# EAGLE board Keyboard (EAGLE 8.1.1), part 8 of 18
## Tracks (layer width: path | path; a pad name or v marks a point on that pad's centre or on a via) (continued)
S$7677 (continued)
  Bottom 0: 271.1,39.77 271.09,39.71
S$7678
  Bottom 0: 271.09,39.71 271.09,39.64
S$7679
  Bottom 0: 271.09,39.64 271.09,38.2
S$7680
  Bottom 0: 271.09,38.2 268.72,38.2
S$7681
  Bottom 0: 268.72,38.2 268.71,38.22
S$7682
  Bottom 0: 268.71,38.22 268.5,38.38
S$7683
  Bottom 0: 268.5,38.38 268.26,38.44
S$7684
  Bottom 0: 268.26,38.44 268.01,38.42
S$7685
  Bottom 0: 268.01,38.42 267.79,38.31
S$7686
  Bottom 0: 267.79,38.31 267.61,38.12
S$7687
  Bottom 0: 267.61,38.12 267.53,37.89
S$7688
  Bottom 0: 267.53,37.89 267.53,37.63
S$7689
  Bottom 0: 267.53,37.63 267.61,37.4
S$7690
  Bottom 0: 267.61,37.4 267.79,37.21
S$7691
  Bottom 0: 267.79,37.21 268.01,37.1
S$7692
  Bottom 0: 268.01,37.1 268.26,37.08
S$7693
  Bottom 0: 268.26,37.08 268.5,37.15
S$7694
  Bottom 0: 268.5,37.15 268.71,37.3
S$7695
  Bottom 0: 268.71,37.3 268.72,37.32
S$7696
  Bottom 0: 268.72,37.32 271.09,37.32
S$7697
  Bottom 0: 271.09,37.32 271.09,15.75
S$7698
  Bottom 0: 271.09,15.75 271.09,15.68
S$7699
  Bottom 0: 271.09,15.68 271.1,15.61
S$7700
  Bottom 0: 271.1,15.61 271.13,15.55
S$7701
  Bottom 0: 271.13,15.55 271.17,15.49
S$7702
  Bottom 0: 271.17,15.49 271.21,15.44
S$7703
  Bottom 0: 271.21,15.44 276.79,9.86
S$7704
  Bottom 0: 276.79,9.86 276.84,9.82
S$7705
  Bottom 0: 276.84,9.82 276.9,9.78
S$7706
  Bottom 0: 276.9,9.78 276.96,9.76
S$7707
  Bottom 0: 276.96,9.76 277.03,9.74
S$7708
  Bottom 0: 277.03,9.74 277.1,9.74
S$7709
  Bottom 0: 277.1,9.74 277.62,9.74
S$7710
  Bottom 0: 277.62,9.74 277.37,9.66
S$7711
  Bottom 0: 277.37,9.66 276.97,9.45
S$7712
  Bottom 0: 276.97,9.45 276.62,9.16
S$7713
  Bottom 0: 276.62,9.16 276.34,8.82
S$7714
  Bottom 0: 276.34,8.82 276.12,8.42
S$7715
  Bottom 0: 276.12,8.42 276,7.99
S$7716
  Bottom 0: 276,7.99 275.95,7.55
S$7717
  Bottom 0: 275.95,7.55 276,7.1
S$7718
  Bottom 0: 276,7.1 276.11,6.75
S$7719
  Bottom 0: 107.77,7.27 107.8,7.43
S$7720
  Bottom 0: 107.8,7.43 107.75,7.75
S$7721
  Bottom 0: 107.75,7.75 107.75,7.78
S$7722
  Bottom 0: 107.75,7.78 107.88,7.9
S$7723
  Bottom 0: 107.88,7.9 107.94,7.97
S$7724
  Bottom 0: 107.94,7.97 107.98,8.04
S$7725
  Bottom 0: 107.98,8.04 108.02,8.12
S$7726
  Bottom 0: 108.02,8.12 108.04,8.21
S$7727
  Bottom 0: 108.04,8.21 108.04,8.3
S$7728
  Bottom 0: 108.04,8.3 108.04,22.57
S$7729
  Bottom 0: 108.04,22.57 108.08,22.6
S$7730
  Bottom 0: 108.08,22.6 110.11,24.64
S$7731
  Bottom 0: 110.11,24.64 110.08,24.58
S$7732
  Bottom 0: 110.08,24.58 109.99,24.24
S$7733
  Bottom 0: 109.99,24.24 109.99,23.89
S$7734
  Bottom 0: 109.99,23.89 110.08,23.55
S$7735
  Bottom 0: 110.08,23.55 110.25,23.24
S$7736
  Bottom 0: 110.25,23.24 110.49,22.99
S$7737
  Bottom 0: 110.49,22.99 110.78,22.8
S$7738
  Bottom 0: 110.78,22.8 110.94,22.75
S$7739
  Bottom 0: 110.94,22.75 110.94,10.43
S$7740
  Bottom 0: 110.94,10.43 107.77,7.27
S$7741
  Bottom 0: 45.16,10.87 45.31,11.02
S$7742
  Bottom 0: 45.31,11.02 45.44,11.29
S$7743
  Bottom 0: 45.44,11.29 45.48,11.6
S$7744
  Bottom 0: 45.48,11.6 45.44,11.89
S$7745
  Bottom 0: 45.44,11.89 45.31,12.17
S$7746
  Bottom 0: 45.31,12.17 45.1,12.39
S$7747
  Bottom 0: 45.1,12.39 44.84,12.54
S$7748
  Bottom 0: 44.84,12.54 44.54,12.61
S$7749
  Bottom 0: 44.54,12.61 44.24,12.59
S$7750
  Bottom 0: 44.24,12.59 44.14,12.55
S$7751
  Bottom 0: 44.14,12.55 43.71,12.99
S$7752
  Bottom 0: 43.71,12.99 43.65,13.03
S$7753
  Bottom 0: 43.65,13.03 43.59,13.07
S$7754
  Bottom 0: 43.59,13.07 43.53,13.09
S$7755
  Bottom 0: 43.53,13.09 43.46,13.11
S$7756
  Bottom 0: 43.46,13.11 43.39,13.11
S$7757
  Bottom 0: 43.39,13.11 37.02,13.11
S$7758
  Bottom 0: 37.02,13.11 36.94,13.11
S$7759
  Bottom 0: 36.94,13.11 36.88,13.09
S$7760
  Bottom 0: 36.88,13.09 36.82,13.07
S$7761
  Bottom 0: 36.82,13.07 36.76,13.03
S$7762
  Bottom 0: 36.76,13.03 36.7,12.99
S$7763
  Bottom 0: 36.7,12.99 36.13,12.42
S$7764
  Bottom 0: 36.13,12.42 36.16,12.64
S$7765
  Bottom 0: 36.16,12.64 36.12,12.96
S$7766
  Bottom 0: 36.12,12.96 35.98,13.26
S$7767
  Bottom 0: 35.98,13.26 35.77,13.5
S$7768
  Bottom 0: 35.77,13.5 35.59,13.62
S$7769
  Bottom 0: 35.59,13.62 35.59,16.83
S$7770
  Bottom 0: 35.59,16.83 53.03,16.83
S$7771
  Bottom 0: 53.03,16.83 52.84,16.64
S$7772
  Bottom 0: 52.84,16.64 52.66,16.36
S$7773
  Bottom 0: 52.66,16.36 52.58,16.05
S$7774
  Bottom 0: 52.58,16.05 52.58,15.72
S$7775
  Bottom 0: 52.58,15.72 52.66,15.41
S$7776
  Bottom 0: 52.66,15.41 52.84,15.14
S$7777
  Bottom 0: 52.84,15.14 53.07,14.91
S$7778
  Bottom 0: 53.07,14.91 53.36,14.77
S$7779
  Bottom 0: 53.36,14.77 53.68,14.7
S$7780
  Bottom 0: 53.68,14.7 54,14.72
S$7781
  Bottom 0: 54,14.72 54.22,14.8
S$7782
  Bottom 0: 54.22,14.8 55.28,13.74
S$7783
  Bottom 0: 55.28,13.74 55.26,13.73
S$7784
  Bottom 0: 55.26,13.73 55.2,13.67
S$7785
  Bottom 0: 55.2,13.67 55.16,13.6
S$7786
  Bottom 0: 55.16,13.6 55.15,13.53
S$7787
  Bottom 0: 55.15,13.53 55.15,11.75
S$7788
  Bottom 0: 55.15,11.75 55.16,11.67
S$7789
  Bottom 0: 55.16,11.67 55.2,11.6
S$7790
  Bottom 0: 55.2,11.6 55.26,11.54
S$7791
  Bottom 0: 55.26,11.54 55.33,11.5
S$7792
  Bottom 0: 55.33,11.5 55.41,11.49
S$7793
  Bottom 0: 55.41,11.49 57.18,11.49
S$7794
  Bottom 0: 57.18,11.49 57.26,11.5
S$7795
  Bottom 0: 57.26,11.5 57.33,11.54
S$7796
  Bottom 0: 57.33,11.54 57.38,11.6
S$7797
  Bottom 0: 57.38,11.6 57.43,11.67
S$7798
  Bottom 0: 57.43,11.67 57.44,11.75
S$7799
  Bottom 0: 57.44,11.75 57.44,13.23
S$7800
  Bottom 0: 57.44,13.23 57.73,12.94
S$7801
  Bottom 0: 57.73,12.94 57.69,12.64
S$7802
  Bottom 0: 57.69,12.64 57.73,12.32
S$7803
  Bottom 0: 57.73,12.32 57.87,12.02
S$7804
  Bottom 0: 57.87,12.02 58.09,11.77
S$7805
  Bottom 0: 58.09,11.77 58.36,11.6
S$7806
  Bottom 0: 58.36,11.6 58.67,11.5
S$7807
  Bottom 0: 58.67,11.5 58.96,11.5
S$7808
  Bottom 0: 58.96,11.5 58.32,10.87
S$7809
  Bottom 0: 58.32,10.87 49.93,10.87
S$7810
  Bottom 0: 49.93,10.87 50.07,11.02
S$7811
  Bottom 0: 50.07,11.02 50.2,11.29
S$7812
  Bottom 0: 50.2,11.29 50.25,11.6
S$7813
  Bottom 0: 50.25,11.6 50.2,11.89
S$7814
  Bottom 0: 50.2,11.89 50.07,12.17
S$7815
  Bottom 0: 50.07,12.17 49.87,12.39
S$7816
  Bottom 0: 49.87,12.39 49.6,12.54
S$7817
  Bottom 0: 49.6,12.54 49.31,12.61
S$7818
  Bottom 0: 49.31,12.61 49,12.59
S$7819
  Bottom 0: 49,12.59 48.73,12.47
S$7820
  Bottom 0: 48.73,12.47 48.49,12.29
S$7821
  Bottom 0: 48.49,12.29 48.32,12.04
S$7822
  Bottom 0: 48.32,12.04 48.23,11.75
S$7823
  Bottom 0: 48.23,11.75 48.23,11.44
S$7824
  Bottom 0: 48.23,11.44 48.32,11.15
S$7825
  Bottom 0: 48.32,11.15 48.49,10.9
S$7826
  Bottom 0: 48.49,10.9 48.53,10.87
S$7827
  Bottom 0: 48.53,10.87 45.16,10.87
S$7828
  Bottom 0: 288.12,10.9 288.22,11.02
S$7829
  Bottom 0: 288.22,11.02 288.35,11.29
S$7830
  Bottom 0: 288.35,11.29 288.4,11.6
S$7831
  Bottom 0: 288.4,11.6 288.35,11.89
S$7832
  Bottom 0: 288.35,11.89 288.22,12.17
S$7833
  Bottom 0: 288.22,12.17 288.02,12.39
S$7834
  Bottom 0: 288.02,12.39 287.75,12.54
S$7835
  Bottom 0: 287.75,12.54 287.46,12.61
S$7836
  Bottom 0: 287.46,12.61 287.15,12.59
S$7837
  Bottom 0: 287.15,12.59 286.98,12.52
S$7838
  Bottom 0: 286.98,12.52 287.69,13.23
S$7839
  Bottom 0: 287.69,13.23 287.75,13.29
S$7840
  Bottom 0: 287.75,13.29 287.8,13.37
S$7841
  Bottom 0: 287.8,13.37 287.83,13.45
S$7842
  Bottom 0: 287.83,13.45 287.85,13.54
S$7843
  Bottom 0: 287.85,13.54 287.86,13.63
S$7844
  Bottom 0: 287.86,13.63 287.86,22.31
S$7845
  Bottom 0: 287.86,22.31 288.06,22.15
S$7846
  Bottom 0: 288.06,22.15 288.34,22.04
S$7847
  Bottom 0: 288.34,22.04 288.64,22.02
S$7848
  Bottom 0: 288.64,22.02 288.89,22.07
S$7849
  Bottom 0: 288.89,22.07 289.77,21.2
S$7850
  Bottom 0: 289.77,21.2 289.83,21.15
S$7851
  Bottom 0: 289.83,21.15 289.88,21.11
S$7852
  Bottom 0: 289.88,21.11 289.95,21.09
S$7853
  Bottom 0: 289.95,21.09 290.01,21.07
S$7854
  Bottom 0: 290.01,21.07 290.09,21.06
S$7855
  Bottom 0: 290.09,21.06 293.43,21.06
S$7856
  Bottom 0: 293.43,21.06 293.45,20.99
S$7857
  Bottom 0: 293.45,20.99 293.63,20.68
S$7858
  Bottom 0: 293.63,20.68 293.87,20.43
S$7859
  Bottom 0: 293.87,20.43 294.16,20.24
S$7860
  Bottom 0: 294.16,20.24 294.49,20.14
S$7861
  Bottom 0: 294.49,20.14 294.84,20.11
S$7862
  Bottom 0: 294.84,20.11 295.14,20.17
S$7863
  Bottom 0: 295.14,20.17 295.25,20.14
S$7864
  Bottom 0: 295.25,20.14 295.6,20.11
S$7865
  Bottom 0: 295.6,20.11 295.71,20.14
S$7866
  Bottom 0: 295.71,20.14 289.45,13.87
S$7867
  Bottom 0: 289.45,13.87 289.4,13.81
S$7868
  Bottom 0: 289.4,13.81 289.36,13.75
S$7869
  Bottom 0: 289.36,13.75 289.34,13.69
S$7870
  Bottom 0: 289.34,13.69 289.32,13.63
S$7871
  Bottom 0: 289.32,13.63 289.32,13.56
S$7872
  Bottom 0: 289.32,13.56 289.32,12.5
S$7873
  Bottom 0: 289.32,12.5 289.25,12.47
S$7874
  Bottom 0: 289.25,12.47 289.01,12.29
S$7875
  Bottom 0: 289.01,12.29 288.85,12.04
S$7876
  Bottom 0: 288.85,12.04 288.75,11.75
S$7877
  Bottom 0: 288.75,11.75 288.75,11.44
S$7878
  Bottom 0: 288.75,11.44 288.85,11.15
S$7879
  Bottom 0: 288.85,11.15 289.01,10.9
S$7880
  Bottom 0: 289.01,10.9 288.12,10.9
S$7881
  Bottom 0: 290.49,10.9 290.6,11.02
S$7882
  Bottom 0: 290.6,11.02 290.73,11.29
S$7883
  Bottom 0: 290.73,11.29 290.78,11.6
S$7884
  Bottom 0: 290.78,11.6 290.73,11.89
S$7885
  Bottom 0: 290.73,11.89 290.6,12.17
S$7886
  Bottom 0: 290.6,12.17 290.4,12.39
S$7887
  Bottom 0: 290.4,12.39 290.2,12.5
S$7888
  Bottom 0: 290.2,12.5 290.2,13.37
S$7889
  Bottom 0: 290.2,13.37 293.19,16.36
S$7890
  Bottom 0: 293.19,16.36 293.11,16.05
S$7891
  Bottom 0: 293.11,16.05 293.11,15.72
S$7892
  Bottom 0: 293.11,15.72 293.19,15.41
S$7893
  Bottom 0: 293.19,15.41 293.37,15.14
S$7894
  Bottom 0: 293.37,15.14 293.6,14.91
S$7895
  Bottom 0: 293.6,14.91 293.89,14.77
S$7896
  Bottom 0: 293.89,14.77 294.21,14.7
S$7897
  Bottom 0: 294.21,14.7 294.53,14.72
S$7898
  Bottom 0: 294.53,14.72 294.57,14.73
S$7899
  Bottom 0: 294.57,14.73 295.52,13.77
S$7900
  Bottom 0: 295.52,13.77 295.13,13.77
S$7901
  Bottom 0: 295.13,13.77 295.06,13.76
S$7902
  Bottom 0: 295.06,13.76 294.99,13.72
S$7903
  Bottom 0: 294.99,13.72 294.93,13.66
S$7904
  Bottom 0: 294.93,13.66 294.89,13.59
S$7905
  Bottom 0: 294.89,13.59 294.88,13.52
S$7906
  Bottom 0: 294.88,13.52 294.88,11.74
S$7907
  Bottom 0: 294.88,11.74 294.89,11.66
S$7908
  Bottom 0: 294.89,11.66 294.93,11.59
S$7909
  Bottom 0: 294.93,11.59 294.99,11.53
S$7910
  Bottom 0: 294.99,11.53 295.06,11.49
S$7911
  Bottom 0: 295.06,11.49 295.13,11.48
S$7912
  Bottom 0: 295.13,11.48 297.19,11.48
S$7913
  Bottom 0: 297.19,11.48 296.61,10.9
S$7914
  Bottom 0: 296.61,10.9 290.49,10.9
S$7915
  Bottom 0: 219.65,11.68 207.87,23.45
S$7916
  Bottom 0: 207.87,23.45 207.98,23.72
S$7917
  Bottom 0: 207.98,23.72 208.02,24.07
S$7918
  Bottom 0: 208.02,24.07 207.98,24.41
S$7919
  Bottom 0: 207.98,24.41 207.87,24.69
S$7920
  Bottom 0: 207.87,24.69 208.32,25.14
S$7921
  Bottom 0: 208.32,25.14 208.36,25.19
S$7922
  Bottom 0: 208.36,25.19 208.4,25.25
S$7923
  Bottom 0: 208.4,25.25 208.43,25.32
S$7924
  Bottom 0: 208.43,25.32 208.44,25.38
S$7925
  Bottom 0: 208.44,25.38 208.45,25.45
S$7926
  Bottom 0: 208.45,25.45 208.45,40.27
S$7927
  Bottom 0: 208.45,40.27 208.5,40.06
S$7928
  Bottom 0: 208.5,40.06 208.67,39.75
S$7929
  Bottom 0: 208.67,39.75 208.91,39.5
S$7930
  Bottom 0: 208.91,39.5 209.21,39.31
S$7931
  Bottom 0: 209.21,39.31 209.54,39.2
S$7932
  Bottom 0: 209.54,39.2 209.89,39.19
S$7933
  Bottom 0: 209.89,39.19 210.23,39.25
S$7934
  Bottom 0: 210.23,39.25 210.55,39.4
S$7935
  Bottom 0: 210.55,39.4 210.82,39.62
S$7936
  Bottom 0: 210.82,39.62 211.03,39.91
S$7937
  Bottom 0: 211.03,39.91 211.15,40.23
S$7938
  Bottom 0: 211.15,40.23 211.2,40.58
S$7939
  Bottom 0: 211.2,40.58 211.15,40.92
S$7940
  Bottom 0: 211.15,40.92 211.03,41.25
S$7941
  Bottom 0: 211.03,41.25 210.82,41.53
S$7942
  Bottom 0: 210.82,41.53 210.55,41.76
S$7943
  Bottom 0: 210.55,41.76 210.23,41.91
S$7944
  Bottom 0: 210.23,41.91 209.89,41.97
S$7945
  Bottom 0: 209.89,41.97 209.54,41.95
S$7946
  Bottom 0: 209.54,41.95 209.21,41.84
S$7947
  Bottom 0: 209.21,41.84 208.91,41.65
S$7948
  Bottom 0: 208.91,41.65 208.67,41.4
S$7949
  Bottom 0: 208.67,41.4 208.5,41.09
S$7950
  Bottom 0: 208.5,41.09 208.45,40.89
S$7951
  Bottom 0: 208.45,40.89 208.45,41.26
S$7952
  Bottom 0: 208.45,41.26 208.44,41.33
S$7953
  Bottom 0: 208.44,41.33 208.43,41.39
S$7954
  Bottom 0: 208.43,41.39 208.4,41.45
S$7955
  Bottom 0: 208.4,41.45 208.36,41.52
S$7956
  Bottom 0: 208.36,41.52 208.32,41.57
S$7957
  Bottom 0: 208.32,41.57 201.82,48.08
S$7958
  Bottom 0: 201.82,48.08 201.83,48.12
S$7959
  Bottom 0: 201.83,48.12 201.78,48.37
S$7960
  Bottom 0: 201.78,48.37 201.65,48.59
S$7961
  Bottom 0: 201.65,48.59 201.45,48.74
S$7962
  Bottom 0: 201.45,48.74 201.21,48.81
S$7963
  Bottom 0: 201.21,48.81 200.96,48.78
S$7964
  Bottom 0: 200.96,48.78 200.73,48.67
S$7965
  Bottom 0: 200.73,48.67 200.56,48.49
S$7966
  Bottom 0: 200.56,48.49 200.47,48.25
S$7967
  Bottom 0: 200.47,48.25 200.47,48.18
S$7968
  Bottom 0: 200.47,48.18 196.29,52.36
S$7969
  Bottom 0: 196.29,52.36 196.79,52.85
S$7970
  Bottom 0: 196.79,52.85 197.04,52.8
S$7971
  Bottom 0: 197.04,52.8 197.37,52.82
S$7972
  Bottom 0: 197.37,52.82 197.67,52.93
S$7973
  Bottom 0: 197.67,52.93 197.94,53.11
S$7974
  Bottom 0: 197.94,53.11 198.14,53.37
S$7975
  Bottom 0: 198.14,53.37 198.27,53.67
S$7976
  Bottom 0: 198.27,53.67 198.32,53.98
S$7977
  Bottom 0: 198.32,53.98 198.27,54.3
S$7978
  Bottom 0: 198.27,54.3 198.14,54.61
S$7979
  Bottom 0: 198.14,54.61 197.94,54.86
S$7980
  Bottom 0: 197.94,54.86 197.67,55.05
S$7981
  Bottom 0: 197.67,55.05 197.37,55.16
S$7982
  Bottom 0: 197.37,55.16 197.04,55.18
S$7983
  Bottom 0: 197.04,55.18 196.72,55.11
S$7984
  Bottom 0: 196.72,55.11 196.43,54.96
S$7985
  Bottom 0: 196.43,54.96 196.2,54.74
S$7986
  Bottom 0: 196.2,54.74 196.02,54.47
S$7987
  Bottom 0: 196.02,54.47 195.94,54.15
S$7988
  Bottom 0: 195.94,54.15 195.94,53.83
S$7989
  Bottom 0: 195.94,53.83 195.98,53.66
S$7990
  Bottom 0: 195.98,53.66 195.25,52.93
S$7991
  Bottom 0: 195.25,52.93 190.05,52.93
S$7992
  Bottom 0: 190.05,52.93 190.31,53.11
S$7993
  Bottom 0: 190.31,53.11 190.52,53.37
S$7994
  Bottom 0: 190.52,53.37 190.65,53.67
S$7995
  Bottom 0: 190.65,53.67 190.7,53.98
S$7996
  Bottom 0: 190.7,53.98 190.65,54.3
S$7997
  Bottom 0: 190.65,54.3 190.52,54.61
S$7998
  Bottom 0: 190.52,54.61 190.31,54.86
S$7999
  Bottom 0: 190.31,54.86 190.05,55.05
S$8000
  Bottom 0: 190.05,55.05 189.75,55.16
S$8001
  Bottom 0: 189.75,55.16 189.42,55.18
S$8002
  Bottom 0: 189.42,55.18 189.1,55.11
S$8003
  Bottom 0: 189.1,55.11 188.81,54.96
S$8004
  Bottom 0: 188.81,54.96 188.58,54.74
S$8005
  Bottom 0: 188.58,54.74 188.41,54.47
S$8006
  Bottom 0: 188.41,54.47 188.32,54.15
S$8007
  Bottom 0: 188.32,54.15 188.32,53.83
S$8008
  Bottom 0: 188.32,53.83 188.41,53.51
S$8009
  Bottom 0: 188.41,53.51 188.58,53.23
S$8010
  Bottom 0: 188.58,53.23 188.81,53.01
S$8011
  Bottom 0: 188.81,53.01 188.98,52.93
S$8012
  Bottom 0: 188.98,52.93 179.94,52.93
S$8013
  Bottom 0: 179.94,52.93 179.22,53.65
S$8014
  Bottom 0: 179.22,53.65 179.22,53.67
S$8015
  Bottom 0: 179.22,53.67 179.27,53.98
S$8016
  Bottom 0: 179.27,53.98 179.22,54.3
S$8017
  Bottom 0: 179.22,54.3 179.09,54.61
S$8018
  Bottom 0: 179.09,54.61 178.88,54.86
S$8019
  Bottom 0: 178.88,54.86 178.62,55.05
S$8020
  Bottom 0: 178.62,55.05 178.32,55.16
S$8021
  Bottom 0: 178.32,55.16 177.99,55.18
S$8022
  Bottom 0: 177.99,55.18 177.67,55.11
S$8023
  Bottom 0: 177.67,55.11 177.38,54.96
S$8024
  Bottom 0: 177.38,54.96 177.15,54.74
S$8025
  Bottom 0: 177.15,54.74 176.97,54.47
S$8026
  Bottom 0: 176.97,54.47 176.89,54.15
S$8027
  Bottom 0: 176.89,54.15 176.89,53.83
S$8028
  Bottom 0: 176.89,53.83 176.97,53.51
S$8029
  Bottom 0: 176.97,53.51 177.15,53.23
S$8030
  Bottom 0: 177.15,53.23 177.38,53.01
S$8031
  Bottom 0: 177.38,53.01 177.67,52.87
S$8032
  Bottom 0: 177.67,52.87 177.99,52.8
S$8033
  Bottom 0: 177.99,52.8 178.32,52.82
S$8034
  Bottom 0: 178.32,52.82 178.41,52.85
S$8035
  Bottom 0: 178.41,52.85 179.14,52.12
S$8036
  Bottom 0: 179.14,52.12 179.14,43.98
S$8037
  Bottom 0: 179.14,43.98 179.07,44.07
S$8038
  Bottom 0: 179.07,44.07 178.8,44.3
S$8039
  Bottom 0: 178.8,44.3 178.49,44.44
S$8040
  Bottom 0: 178.49,44.44 178.49,50.68
S$8041
  Bottom 0: 178.49,50.68 178.49,50.75
S$8042
  Bottom 0: 178.49,50.75 178.47,50.81
S$8043
  Bottom 0: 178.47,50.81 178.45,50.87
S$8044
  Bottom 0: 178.45,50.87 178.41,50.94
S$8045
  Bottom 0: 178.41,50.94 178.37,50.99
S$8046
  Bottom 0: 178.37,50.99 173.39,55.96
S$8047
  Bottom 0: 173.39,55.96 173.4,56.01
S$8048
  Bottom 0: 173.4,56.01 173.36,56.26
S$8049
  Bottom 0: 173.36,56.26 173.22,56.47
S$8050
  Bottom 0: 173.22,56.47 173.02,56.62
S$8051
  Bottom 0: 173.02,56.62 172.78,56.69
S$8052
  Bottom 0: 172.78,56.69 172.53,56.67
S$8053
  Bottom 0: 172.53,56.67 172.3,56.56
S$8054
  Bottom 0: 172.3,56.56 172.13,56.37
S$8055
  Bottom 0: 172.13,56.37 172.04,56.14
S$8056
  Bottom 0: 172.04,56.14 172.04,55.88
S$8057
  Bottom 0: 172.04,55.88 172.13,55.65
S$8058
  Bottom 0: 172.13,55.65 172.3,55.46
S$8059
  Bottom 0: 172.3,55.46 172.53,55.35
S$8060
  Bottom 0: 172.53,55.35 172.77,55.33
S$8061
  Bottom 0: 172.77,55.33 177.61,50.49
S$8062
  Bottom 0: 177.61,50.49 177.61,44.43
S$8063
  Bottom 0: 177.61,44.43 177.46,44.38
S$8064
  Bottom 0: 177.46,44.38 177.16,44.19
S$8065
  Bottom 0: 177.16,44.19 176.92,43.94
S$8066
  Bottom 0: 176.92,43.94 176.75,43.63
S$8067
  Bottom 0: 176.75,43.63 176.66,43.29
S$8068
  Bottom 0: 176.66,43.29 176.66,42.94
S$8069
  Bottom 0: 176.66,42.94 176.75,42.6
S$8070
  Bottom 0: 176.75,42.6 176.92,42.29
S$8071
  Bottom 0: 176.92,42.29 177.16,42.04
S$8072
  Bottom 0: 177.16,42.04 177.46,41.85
S$8073
  Bottom 0: 177.46,41.85 177.79,41.74
S$8074
  Bottom 0: 177.79,41.74 178.14,41.73
S$8075
  Bottom 0: 178.14,41.73 178.48,41.79
S$8076
  Bottom 0: 178.48,41.79 178.8,41.94
S$8077
  Bottom 0: 178.8,41.94 179.07,42.16
S$8078
  Bottom 0: 179.07,42.16 179.14,42.26
S$8079
  Bottom 0: 179.14,42.26 179.14,38.13
S$8080
  Bottom 0: 179.14,38.13 178.01,37.01
S$8081
  Bottom 0: 178.01,37.01 177.94,36.94
S$8082
  Bottom 0: 177.94,36.94 177.9,36.86
S$8083
  Bottom 0: 177.9,36.86 177.87,36.78
S$8084
  Bottom 0: 177.87,36.78 177.84,36.7
S$8085
  Bottom 0: 177.84,36.7 177.84,36.6
S$8086
  Bottom 0: 177.84,36.6 177.84,33.64
S$8087
  Bottom 0: 177.84,33.64 170.65,33.64
S$8088
  Bottom 0: 170.65,33.64 169.69,34.6
S$8089
  Bottom 0: 169.69,34.6 169.69,34.62
S$8090
  Bottom 0: 169.69,34.62 169.74,34.94
S$8091
  Bottom 0: 169.74,34.94 169.69,35.26
S$8092
  Bottom 0: 169.69,35.26 169.56,35.56
S$8093
  Bottom 0: 169.56,35.56 169.36,35.81
S$8094
  Bottom 0: 169.36,35.81 169.09,36
S$8095
  Bottom 0: 169.09,36 168.79,36.11
S$8096
  Bottom 0: 168.79,36.11 168.47,36.13
S$8097
  Bottom 0: 168.47,36.13 168.15,36.06
S$8098
  Bottom 0: 168.15,36.06 168.01,35.99
S$8099
  Bottom 0: 168.01,35.99 161.34,42.66
S$8100
  Bottom 0: 161.34,42.66 161.34,52.24
S$8101
  Bottom 0: 161.34,52.24 161.33,52.33
S$8102
  Bottom 0: 161.33,52.33 161.31,52.42
S$8103
  Bottom 0: 161.31,52.42 161.28,52.5
S$8104
  Bottom 0: 161.28,52.5 161.23,52.58
S$8105
  Bottom 0: 161.23,52.58 161.17,52.65
S$8106
  Bottom 0: 161.17,52.65 160.16,53.65
S$8107
  Bottom 0: 160.16,53.65 160.17,53.67
S$8108
  Bottom 0: 160.17,53.67 160.22,53.99
S$8109
  Bottom 0: 160.22,53.99 160.17,54.31
S$8110
  Bottom 0: 160.17,54.31 160.04,54.61
S$8111
  Bottom 0: 160.04,54.61 159.84,54.87
S$8112
  Bottom 0: 159.84,54.87 159.57,55.05
S$8113
  Bottom 0: 159.57,55.05 159.27,55.16
S$8114
  Bottom 0: 159.27,55.16 158.94,55.18
S$8115
  Bottom 0: 158.94,55.18 158.62,55.12
S$8116
  Bottom 0: 158.62,55.12 158.33,54.97
S$8117
  Bottom 0: 158.33,54.97 158.09,54.74
S$8118
  Bottom 0: 158.09,54.74 157.92,54.47
S$8119
  Bottom 0: 157.92,54.47 157.84,54.16
S$8120
  Bottom 0: 157.84,54.16 157.84,53.83
S$8121
  Bottom 0: 157.84,53.83 157.92,53.52
S$8122
  Bottom 0: 157.92,53.52 158.09,53.24
S$8123
  Bottom 0: 158.09,53.24 158.33,53.02
S$8124
  Bottom 0: 158.33,53.02 158.62,52.87
S$8125
  Bottom 0: 158.62,52.87 158.94,52.8
S$8126
  Bottom 0: 158.94,52.8 159.27,52.82
S$8127
  Bottom 0: 159.27,52.82 159.36,52.85
S$8128
  Bottom 0: 159.36,52.85 160.2,52.01
S$8129
  Bottom 0: 160.2,52.01 160.2,43.82
S$8130
  Bottom 0: 160.2,43.82 160.02,44.07
S$8131
  Bottom 0: 160.02,44.07 159.75,44.3
S$8132
  Bottom 0: 159.75,44.3 159.44,44.44
S$8133
  Bottom 0: 159.44,44.44 159.44,51.54
S$8134
  Bottom 0: 159.44,51.54 159.44,51.61
S$8135
  Bottom 0: 159.44,51.61 159.42,51.68
S$8136
  Bottom 0: 159.42,51.68 159.4,51.74
S$8137
  Bottom 0: 159.4,51.74 159.36,51.8
S$8138
  Bottom 0: 159.36,51.8 159.31,51.85
S$8139
  Bottom 0: 159.31,51.85 156.04,55.12
S$8140
  Bottom 0: 156.04,55.12 156.06,55.17
S$8141
  Bottom 0: 156.06,55.17 156.01,55.41
S$8142
  Bottom 0: 156.01,55.41 155.88,55.63
S$8143
  Bottom 0: 155.88,55.63 155.67,55.78
S$8144
  Bottom 0: 155.67,55.78 155.43,55.85
S$8145
  Bottom 0: 155.43,55.85 155.18,55.83
S$8146
  Bottom 0: 155.18,55.83 154.96,55.72
S$8147
  Bottom 0: 154.96,55.72 154.92,55.67
S$8148
  Bottom 0: 154.92,55.67 154.92,56.04
S$8149
  Bottom 0: 154.92,56.04 156.43,57.54
S$8150
  Bottom 0: 156.43,57.54 169.11,57.54
S$8151
  Bottom 0: 169.11,57.54 169.18,57.55
S$8152
  Bottom 0: 169.18,57.55 169.25,57.56
S$8153
  Bottom 0: 169.25,57.56 169.31,57.59
S$8154
  Bottom 0: 169.31,57.59 169.37,57.63
S$8155
  Bottom 0: 169.37,57.63 169.43,57.67
S$8156
  Bottom 0: 169.43,57.67 172.67,60.92
S$8157
  Bottom 0: 172.67,60.92 172.7,60.9
S$8158
  Bottom 0: 172.7,60.9 173.03,60.8
S$8159
  Bottom 0: 173.03,60.8 173.38,60.77
S$8160
  Bottom 0: 173.38,60.77 173.72,60.84
S$8161
  Bottom 0: 173.72,60.84 173.91,60.93
S$8162
  Bottom 0: 173.91,60.93 178.11,56.72
S$8163
  Bottom 0: 178.11,56.72 178.16,56.67
S$8164
  Bottom 0: 178.16,56.67 178.22,56.63
S$8165
  Bottom 0: 178.22,56.63 178.28,56.61
S$8166
  Bottom 0: 178.28,56.61 178.35,56.59
S$8167
  Bottom 0: 178.35,56.59 178.42,56.59
S$8168
  Bottom 0: 178.42,56.59 197.17,56.59
S$8169
  Bottom 0: 197.17,56.59 203.09,50.67
S$8170
  Bottom 0: 203.09,50.67 202.91,50.71
S$8171
  Bottom 0: 202.91,50.71 202.61,50.69
S$8172
  Bottom 0: 202.61,50.69 202.33,50.58
S$8173
  Bottom 0: 202.33,50.58 202.09,50.39
S$8174
  Bottom 0: 202.09,50.39 201.92,50.14
S$8175
  Bottom 0: 201.92,50.14 201.83,49.85
S$8176
  Bottom 0: 201.83,49.85 201.83,49.55
S$8177
  Bottom 0: 201.83,49.55 201.92,49.26
S$8178
  Bottom 0: 201.92,49.26 202.09,49.01
S$8179
  Bottom 0: 202.09,49.01 202.33,48.82
S$8180
  Bottom 0: 202.33,48.82 202.61,48.71
S$8181
  Bottom 0: 202.61,48.71 202.91,48.69
S$8182
  Bottom 0: 202.91,48.69 203.21,48.76
S$8183
  Bottom 0: 203.21,48.76 203.47,48.91
S$8184
  Bottom 0: 203.47,48.91 203.67,49.13
S$8185
  Bottom 0: 203.67,49.13 203.81,49.4
S$8186
  Bottom 0: 203.81,49.4 203.85,49.7
S$8187
  Bottom 0: 203.85,49.7 203.81,49.95
S$8188
  Bottom 0: 203.81,49.95 206.02,47.74
S$8189
  Bottom 0: 206.02,47.74 206.08,47.7
S$8190
  Bottom 0: 206.08,47.7 206.14,47.66
S$8191
  Bottom 0: 206.14,47.66 206.2,47.63
S$8192
  Bottom 0: 206.2,47.63 206.27,47.62
S$8193
  Bottom 0: 206.27,47.62 206.33,47.62
S$8194
  Bottom 0: 206.33,47.62 211.18,47.62
S$8195
  Bottom 0: 211.18,47.62 211.07,47.56
S$8196
  Bottom 0: 211.07,47.56 210.73,47.27
S$8197
  Bottom 0: 210.73,47.27 210.44,46.93
S$8198
  Bottom 0: 210.44,46.93 210.23,46.53
S$8199
  Bottom 0: 210.23,46.53 210.1,46.1
S$8200
  Bottom 0: 210.1,46.1 210.06,45.66
S$8201
  Bottom 0: 210.06,45.66 210.1,45.21
S$8202
  Bottom 0: 210.1,45.21 210.23,44.78
S$8203
  Bottom 0: 210.23,44.78 210.44,44.39
S$8204
  Bottom 0: 210.44,44.39 210.73,44.04
S$8205
  Bottom 0: 210.73,44.04 211.07,43.76
S$8206
  Bottom 0: 211.07,43.76 211.47,43.54
S$8207
  Bottom 0: 211.47,43.54 211.89,43.42
S$8208
  Bottom 0: 211.89,43.42 212.34,43.37
S$8209
  Bottom 0: 212.34,43.37 212.79,43.42
S$8210
  Bottom 0: 212.79,43.42 213.22,43.54
S$8211
  Bottom 0: 213.22,43.54 213.61,43.76
S$8212
  Bottom 0: 213.61,43.76 213.95,44.04
S$8213
  Bottom 0: 213.95,44.04 214.24,44.39
S$8214
  Bottom 0: 214.24,44.39 214.46,44.78
S$8215
  Bottom 0: 214.46,44.78 214.58,45.21
S$8216
  Bottom 0: 214.58,45.21 214.63,45.66
S$8217
  Bottom 0: 214.63,45.66 214.58,46.1
S$8218
  Bottom 0: 214.58,46.1 214.55,46.22
S$8219
  Bottom 0: 214.55,46.22 215.71,45.06
S$8220
  Bottom 0: 215.71,45.06 215.71,44.43
S$8221
  Bottom 0: 215.71,44.43 215.56,44.38
S$8222
  Bottom 0: 215.56,44.38 215.26,44.19
S$8223
  Bottom 0: 215.26,44.19 215.02,43.94
S$8224
  Bottom 0: 215.02,43.94 214.85,43.63
S$8225
  Bottom 0: 214.85,43.63 214.76,43.29
S$8226
  Bottom 0: 214.76,43.29 214.76,42.94
S$8227
  Bottom 0: 214.76,42.94 214.85,42.6
S$8228
  Bottom 0: 214.85,42.6 215.02,42.29
S$8229
  Bottom 0: 215.02,42.29 215.26,42.04
S$8230
  Bottom 0: 215.26,42.04 215.56,41.85
S$8231
  Bottom 0: 215.56,41.85 215.89,41.74
S$8232
  Bottom 0: 215.89,41.74 216.24,41.73
S$8233
  Bottom 0: 216.24,41.73 216.58,41.79
S$8234
  Bottom 0: 216.58,41.79 216.9,41.94
S$8235
  Bottom 0: 216.9,41.94 217.17,42.16
S$8236
  Bottom 0: 217.17,42.16 217.38,42.45
S$8237
  Bottom 0: 217.38,42.45 217.5,42.77
S$8238
  Bottom 0: 217.5,42.77 217.55,43.12
S$8239
  Bottom 0: 217.55,43.12 217.5,43.46
S$8240
  Bottom 0: 217.5,43.46 217.49,43.5
S$8241
  Bottom 0: 217.49,43.5 222.42,38.57
S$8242
  Bottom 0: 222.42,38.57 222.42,32.57
S$8243
  Bottom 0: 222.42,32.57 222.39,32.55
S$8244
  Bottom 0: 222.39,32.55 222.18,32.31
S$8245
  Bottom 0: 222.18,32.31 222.04,32.01
S$8246
  Bottom 0: 222.04,32.01 221.99,31.69
S$8247
  Bottom 0: 221.99,31.69 222.03,31.39
S$8248
  Bottom 0: 222.03,31.39 221.74,31.1
S$8249
  Bottom 0: 221.74,31.1 221.74,32.58
S$8250
  Bottom 0: 221.74,32.58 221.73,32.65
S$8251
  Bottom 0: 221.73,32.65 221.69,32.72
S$8252
  Bottom 0: 221.69,32.72 221.63,32.78
S$8253
  Bottom 0: 221.63,32.78 221.56,32.82
S$8254
  Bottom 0: 221.56,32.82 221.49,32.83
S$8255
  Bottom 0: 221.49,32.83 221.04,32.83
S$8256
  Bottom 0: 221.04,32.83 221.04,32.96
S$8257
  Bottom 0: 221.04,32.96 220.98,33.18
S$8258
  Bottom 0: 220.98,33.18 220.81,33.34
S$8259
  Bottom 0: 220.81,33.34 220.6,33.4
S$8260
  Bottom 0: 220.6,33.4 220.25,33.4
S$8261
  Bottom 0: 220.25,33.4 219.17,34.48
S$8262
  Bottom 0: 219.17,34.48 219.23,34.62
S$8263
  Bottom 0: 219.23,34.62 219.28,34.94
S$8264
  Bottom 0: 219.28,34.94 219.23,35.26
S$8265
  Bottom 0: 219.23,35.26 219.1,35.56
S$8266
  Bottom 0: 219.1,35.56 218.9,35.81
S$8267
  Bottom 0: 218.9,35.81 218.63,36
S$8268
  Bottom 0: 218.63,36 218.33,36.11
S$8269
  Bottom 0: 218.33,36.11 218,36.13
S$8270
  Bottom 0: 218,36.13 217.68,36.06
S$8271
  Bottom 0: 217.68,36.06 217.39,35.91
S$8272
  Bottom 0: 217.39,35.91 217.16,35.69
S$8273
  Bottom 0: 217.16,35.69 216.99,35.41
S$8274
  Bottom 0: 216.99,35.41 216.9,35.1
S$8275
  Bottom 0: 216.9,35.1 216.9,34.77
S$8276
  Bottom 0: 216.9,34.77 216.99,34.46
S$8277
  Bottom 0: 216.99,34.46 217.16,34.19
S$8278
  Bottom 0: 217.16,34.19 217.39,33.96
S$8279
  Bottom 0: 217.39,33.96 217.68,33.81
S$8280
  Bottom 0: 217.68,33.81 218,33.75
S$8281
  Bottom 0: 218,33.75 218.33,33.77
S$8282
  Bottom 0: 218.33,33.77 218.54,33.85
S$8283
  Bottom 0: 218.54,33.85 219.59,32.8
S$8284
  Bottom 0: 219.59,32.8 219.56,32.78
S$8285
  Bottom 0: 219.56,32.78 219.5,32.72
S$8286
  Bottom 0: 219.5,32.72 219.46,32.65
S$8287
  Bottom 0: 219.46,32.65 219.45,32.58
S$8288
  Bottom 0: 219.45,32.58 219.45,30.8
S$8289
  Bottom 0: 219.45,30.8 219.46,30.72
S$8290
  Bottom 0: 219.46,30.72 219.5,30.65
S$8291
  Bottom 0: 219.5,30.65 219.56,30.59
S$8292
  Bottom 0: 219.56,30.59 219.63,30.55
S$8293
  Bottom 0: 219.63,30.55 219.71,30.54
S$8294
  Bottom 0: 219.71,30.54 221.19,30.54
S$8295
  Bottom 0: 221.19,30.54 217.26,26.61
S$8296
  Bottom 0: 217.26,26.61 217.19,26.55
S$8297
  Bottom 0: 217.19,26.55 217.15,26.47
S$8298
  Bottom 0: 217.15,26.47 217.12,26.39
S$8299
  Bottom 0: 217.12,26.39 217.1,26.3
S$8300
  Bottom 0: 217.1,26.3 217.09,26.21
S$8301
  Bottom 0: 217.09,26.21 217.09,20.55
S$8302
  Bottom 0: 217.09,20.55 217.1,20.46
S$8303
  Bottom 0: 217.1,20.46 217.12,20.37
S$8304
  Bottom 0: 217.12,20.37 217.15,20.29
S$8305
  Bottom 0: 217.15,20.29 217.19,20.22
S$8306
  Bottom 0: 217.19,20.22 217.26,20.15
S$8307
  Bottom 0: 217.26,20.15 218.27,19.13
S$8308
  Bottom 0: 218.27,19.13 218.33,19.08
S$8309
  Bottom 0: 218.33,19.08 218.41,19.03
S$8310
  Bottom 0: 218.41,19.03 218.49,19
S$8311
  Bottom 0: 218.49,19 218.58,18.97
S$8312
  Bottom 0: 218.58,18.97 218.67,18.97
S$8313
  Bottom 0: 218.67,18.97 218.77,18.97
S$8314
  Bottom 0: 218.77,18.97 220.68,17.06
S$8315
  Bottom 0: 220.68,17.06 220.38,17.08
S$8316
  Bottom 0: 220.38,17.08 220.06,17.01
S$8317
  Bottom 0: 220.06,17.01 219.77,16.86
S$8318
  Bottom 0: 219.77,16.86 219.54,16.64
S$8319
  Bottom 0: 219.54,16.64 219.37,16.36
S$8320
  Bottom 0: 219.37,16.36 219.28,16.05
S$8321
  Bottom 0: 219.28,16.05 219.28,15.72
S$8322
  Bottom 0: 219.28,15.72 219.37,15.41
S$8323
  Bottom 0: 219.37,15.41 219.54,15.14
S$8324
  Bottom 0: 219.54,15.14 219.77,14.91
S$8325
  Bottom 0: 219.77,14.91 220.06,14.77
S$8326
  Bottom 0: 220.06,14.77 220.38,14.7
S$8327
  Bottom 0: 220.38,14.7 220.71,14.72
S$8328
  Bottom 0: 220.71,14.72 220.93,14.8
S$8329
  Bottom 0: 220.93,14.8 221.97,13.75
S$8330
  Bottom 0: 221.97,13.75 221.94,13.73
S$8331
  Bottom 0: 221.94,13.73 221.89,13.67
S$8332
  Bottom 0: 221.89,13.67 221.85,13.6
S$8333
  Bottom 0: 221.85,13.6 221.83,13.53
S$8334
  Bottom 0: 221.83,13.53 221.83,11.75
S$8335
  Bottom 0: 221.83,11.75 221.85,11.68
S$8336
  Bottom 0: 221.85,11.68 219.65,11.68
S$8337
  Bottom 0: 212.44,22.02 212.73,22.09
S$8338
  Bottom 0: 212.73,22.09 213,22.24
S$8339
  Bottom 0: 213,22.24 213.2,22.46
S$8340
  Bottom 0: 213.2,22.46 213.33,22.73
S$8341
  Bottom 0: 213.33,22.73 213.38,23.03
S$8342
  Bottom 0: 213.38,23.03 213.33,23.33
S$8343
  Bottom 0: 213.33,23.33 213.2,23.6
S$8344
  Bottom 0: 213.2,23.6 213,23.82
S$8345
  Bottom 0: 213,23.82 212.73,23.98
S$8346
  Bottom 0: 212.73,23.98 212.44,24.04
S$8347
  Bottom 0: 212.44,24.04 212.13,24.02
S$8348
  Bottom 0: 212.13,24.02 211.85,23.91
S$8349
  Bottom 0: 211.85,23.91 211.62,23.72
S$8350
  Bottom 0: 211.62,23.72 211.45,23.47
S$8351
  Bottom 0: 211.45,23.47 211.35,23.18
S$8352
  Bottom 0: 211.35,23.18 211.35,22.88
S$8353
  Bottom 0: 211.35,22.88 211.45,22.59
S$8354
  Bottom 0: 211.45,22.59 211.62,22.34
S$8355
  Bottom 0: 211.62,22.34 211.85,22.15
S$8356
  Bottom 0: 211.85,22.15 212.13,22.04
S$8357
  Bottom 0: 212.13,22.04 212.44,22.02
S$8358
  Bottom 0: 212.44,29.64 212.73,29.7
S$8359
  Bottom 0: 212.73,29.7 213,29.86
S$8360
  Bottom 0: 213,29.86 213.2,30.08
S$8361
  Bottom 0: 213.2,30.08 213.33,30.35
S$8362
  Bottom 0: 213.33,30.35 213.38,30.65
S$8363
  Bottom 0: 213.38,30.65 213.33,30.95
S$8364
  Bottom 0: 213.33,30.95 213.2,31.22
S$8365
  Bottom 0: 213.2,31.22 213,31.44
S$8366
  Bottom 0: 213,31.44 212.73,31.59
S$8367
  Bottom 0: 212.73,31.59 212.44,31.66
S$8368
  Bottom 0: 212.44,31.66 212.13,31.64
S$8369
  Bottom 0: 212.13,31.64 211.85,31.53
S$8370
  Bottom 0: 211.85,31.53 211.62,31.34
S$8371
  Bottom 0: 211.62,31.34 211.45,31.09
S$8372
  Bottom 0: 211.45,31.09 211.35,30.8
S$8373
  Bottom 0: 211.35,30.8 211.35,30.5
S$8374
  Bottom 0: 211.35,30.5 211.45,30.21
S$8375
  Bottom 0: 211.45,30.21 211.62,29.96
S$8376
  Bottom 0: 211.62,29.96 211.85,29.77
S$8377
  Bottom 0: 211.85,29.77 212.13,29.66
S$8378
  Bottom 0: 212.13,29.66 212.44,29.64
S$8379
  Bottom 0: 171.79,39.19 172.13,39.25
S$8380
  Bottom 0: 172.13,39.25 172.45,39.4
S$8381
  Bottom 0: 172.45,39.4 172.72,39.62
S$8382
  Bottom 0: 172.72,39.62 172.93,39.91
S$8383
  Bottom 0: 172.93,39.91 173.05,40.23
S$8384
  Bottom 0: 173.05,40.23 173.1,40.58
S$8385
  Bottom 0: 173.1,40.58 173.05,40.92
S$8386
  Bottom 0: 173.05,40.92 172.93,41.25
S$8387
  Bottom 0: 172.93,41.25 172.72,41.53
S$8388
  Bottom 0: 172.72,41.53 172.45,41.76
S$8389
  Bottom 0: 172.45,41.76 172.13,41.91
S$8390
  Bottom 0: 172.13,41.91 171.79,41.97
S$8391
  Bottom 0: 171.79,41.97 171.44,41.95
S$8392
  Bottom 0: 171.44,41.95 171.11,41.84
S$8393
  Bottom 0: 171.11,41.84 171.08,41.83
S$8394
  Bottom 0: 171.08,41.83 170.51,42.4
S$8395
  Bottom 0: 170.51,42.4 170.45,42.43
S$8396
  Bottom 0: 170.45,42.43 170.39,42.48
S$8397
  Bottom 0: 170.39,42.48 170.33,42.5
S$8398
  Bottom 0: 170.33,42.5 170.27,42.52
S$8399
  Bottom 0: 170.27,42.52 170.2,42.52
S$8400
  Bottom 0: 170.2,42.52 165.64,42.52
S$8401
  Bottom 0: 165.64,42.52 165.57,42.65
S$8402
  Bottom 0: 165.57,42.65 165.37,42.87
S$8403
  Bottom 0: 165.37,42.87 165.11,43.02
S$8404
  Bottom 0: 165.11,43.02 164.81,43.09
S$8405
  Bottom 0: 164.81,43.09 164.51,43.07
S$8406
  Bottom 0: 164.51,43.07 164.23,42.96
S$8407
  Bottom 0: 164.23,42.96 163.99,42.77
S$8408
  Bottom 0: 163.99,42.77 163.82,42.52
S$8409
  Bottom 0: 163.82,42.52 163.73,42.23
S$8410
  Bottom 0: 163.73,42.23 163.73,41.92
S$8411
  Bottom 0: 163.73,41.92 163.82,41.64
S$8412
  Bottom 0: 163.82,41.64 163.99,41.39
S$8413
  Bottom 0: 163.99,41.39 164.23,41.2
S$8414
  Bottom 0: 164.23,41.2 164.51,41.09
S$8415
  Bottom 0: 164.51,41.09 164.81,41.07
S$8416
  Bottom 0: 164.81,41.07 165.11,41.13
S$8417
  Bottom 0: 165.11,41.13 165.37,41.28
S$8418
  Bottom 0: 165.37,41.28 165.57,41.51
S$8419
  Bottom 0: 165.57,41.51 165.64,41.64
S$8420
  Bottom 0: 165.64,41.64 170.01,41.64
S$8421
  Bottom 0: 170.01,41.64 170.45,41.19
S$8422
  Bottom 0: 170.45,41.19 170.4,41.09
S$8423
  Bottom 0: 170.4,41.09 170.31,40.75
S$8424
  Bottom 0: 170.31,40.75 170.31,40.4
S$8425
  Bottom 0: 170.31,40.4 170.4,40.06
S$8426
  Bottom 0: 170.4,40.06 170.57,39.75
S$8427
  Bottom 0: 170.57,39.75 170.81,39.5
S$8428
  Bottom 0: 170.81,39.5 171.11,39.31
S$8429
  Bottom 0: 171.11,39.31 171.44,39.2
S$8430
  Bottom 0: 171.44,39.2 171.79,39.19
S$8431
  Bottom 0: 174.24,43.37 174.69,43.42
S$8432
  Bottom 0: 174.69,43.42 175.12,43.54
S$8433
  Bottom 0: 175.12,43.54 175.51,43.76
S$8434
  Bottom 0: 175.51,43.76 175.85,44.04
S$8435
  Bottom 0: 175.85,44.04 176.14,44.39
S$8436
  Bottom 0: 176.14,44.39 176.35,44.78
S$8437
  Bottom 0: 176.35,44.78 176.48,45.21
S$8438
  Bottom 0: 176.48,45.21 176.53,45.66
S$8439
  Bottom 0: 176.53,45.66 176.48,46.1
S$8440
  Bottom 0: 176.48,46.1 176.35,46.53
S$8441
  Bottom 0: 176.35,46.53 176.14,46.93
S$8442
  Bottom 0: 176.14,46.93 175.85,47.27
S$8443
  Bottom 0: 175.85,47.27 175.51,47.56
S$8444
  Bottom 0: 175.51,47.56 175.12,47.77
S$8445
  Bottom 0: 175.12,47.77 174.69,47.89
S$8446
  Bottom 0: 174.69,47.89 174.24,47.94
S$8447
  Bottom 0: 174.24,47.94 173.79,47.89
S$8448
  Bottom 0: 173.79,47.89 173.37,47.77
S$8449
  Bottom 0: 173.37,47.77 172.97,47.56
S$8450
  Bottom 0: 172.97,47.56 172.63,47.27
S$8451
  Bottom 0: 172.63,47.27 172.34,46.93
S$8452
  Bottom 0: 172.34,46.93 172.13,46.53
S$8453
  Bottom 0: 172.13,46.53 172,46.1
S$8454
  Bottom 0: 172,46.1 171.96,45.66
S$8455
  Bottom 0: 171.96,45.66 172,45.21
S$8456
  Bottom 0: 172,45.21 172.13,44.78
S$8457
  Bottom 0: 172.13,44.78 172.34,44.39
S$8458
  Bottom 0: 172.34,44.39 172.63,44.04
S$8459
  Bottom 0: 172.63,44.04 172.97,43.76
S$8460
  Bottom 0: 172.97,43.76 173.37,43.54
S$8461
  Bottom 0: 173.37,43.54 173.79,43.42
S$8462
  Bottom 0: 173.79,43.42 174.24,43.37
S$8463
  Bottom 0: 164.81,48.69 165.11,48.76
S$8464
  Bottom 0: 165.11,48.76 165.37,48.91
S$8465
  Bottom 0: 165.37,48.91 165.57,49.13
S$8466
  Bottom 0: 165.57,49.13 165.71,49.4
S$8467
  Bottom 0: 165.71,49.4 165.75,49.7
S$8468
  Bottom 0: 165.75,49.7 165.71,50
S$8469
  Bottom 0: 165.71,50 165.57,50.27
S$8470
  Bottom 0: 165.57,50.27 165.37,50.49
S$8471
  Bottom 0: 165.37,50.49 165.11,50.65
S$8472
  Bottom 0: 165.11,50.65 164.81,50.71
S$8473
  Bottom 0: 164.81,50.71 164.51,50.69
S$8474
  Bottom 0: 164.51,50.69 164.23,50.58
S$8475
  Bottom 0: 164.23,50.58 163.99,50.39
S$8476
  Bottom 0: 163.99,50.39 163.82,50.14
S$8477
  Bottom 0: 163.82,50.14 163.73,49.85
S$8478
  Bottom 0: 163.73,49.85 163.73,49.55
S$8479
  Bottom 0: 163.73,49.55 163.82,49.26
S$8480
  Bottom 0: 163.82,49.26 163.99,49.01
S$8481
  Bottom 0: 163.99,49.01 164.23,48.82
S$8482
  Bottom 0: 164.23,48.82 164.51,48.71
S$8483
  Bottom 0: 164.51,48.71 164.81,48.69
S$8484
  Bottom 0: 172.08,49.59 173.86,49.59
S$8485
  Bottom 0: 173.86,49.59 173.94,49.6
S$8486
  Bottom 0: 173.94,49.6 174.01,49.64
S$8487
  Bottom 0: 174.01,49.64 174.06,49.7
S$8488
  Bottom 0: 174.06,49.7 174.1,49.77
S$8489
  Bottom 0: 174.1,49.77 174.11,49.85
S$8490
  Bottom 0: 174.11,49.85 174.11,51.63
S$8491
  Bottom 0: 174.11,51.63 174.1,51.7
S$8492
  Bottom 0: 174.1,51.7 174.06,51.77
S$8493
  Bottom 0: 174.06,51.77 174.01,51.83
S$8494
  Bottom 0: 174.01,51.83 173.94,51.87
S$8495
  Bottom 0: 173.94,51.87 173.86,51.88
S$8496
  Bottom 0: 173.86,51.88 173.41,51.88
S$8497
  Bottom 0: 173.41,51.88 173.41,52.01
S$8498
  Bottom 0: 173.41,52.01 173.35,52.23
S$8499
  Bottom 0: 173.35,52.23 173.19,52.39
S$8500
  Bottom 0: 173.19,52.39 172.97,52.45
S$8501
  Bottom 0: 172.97,52.45 172.62,52.45
S$8502
  Bottom 0: 172.62,52.45 171.54,53.52
S$8503
  Bottom 0: 171.54,53.52 171.6,53.67
S$8504
  Bottom 0: 171.6,53.67 171.65,53.98
S$8505
  Bottom 0: 171.65,53.98 171.6,54.3
S$8506
  Bottom 0: 171.6,54.3 171.47,54.61
S$8507
  Bottom 0: 171.47,54.61 171.26,54.86
S$8508
  Bottom 0: 171.26,54.86 171,55.05
S$8509
  Bottom 0: 171,55.05 170.7,55.16
S$8510
  Bottom 0: 170.7,55.16 170.37,55.18
S$8511
  Bottom 0: 170.37,55.18 170.05,55.11
S$8512
  Bottom 0: 170.05,55.11 169.76,54.96
S$8513
  Bottom 0: 169.76,54.96 169.53,54.74
S$8514
  Bottom 0: 169.53,54.74 169.35,54.47
S$8515
  Bottom 0: 169.35,54.47 169.27,54.15
S$8516
  Bottom 0: 169.27,54.15 169.27,53.83
S$8517
  Bottom 0: 169.27,53.83 169.35,53.51
S$8518
  Bottom 0: 169.35,53.51 169.53,53.23
S$8519
  Bottom 0: 169.53,53.23 169.76,53.01
S$8520
  Bottom 0: 169.76,53.01 170.05,52.87
S$8521
  Bottom 0: 170.05,52.87 170.37,52.8
S$8522
  Bottom 0: 170.37,52.8 170.7,52.82
S$8523
  Bottom 0: 170.7,52.82 170.92,52.9
S$8524
  Bottom 0: 170.92,52.9 171.97,51.85
S$8525
  Bottom 0: 171.97,51.85 171.94,51.83
S$8526
  Bottom 0: 171.94,51.83 171.88,51.77
S$8527
  Bottom 0: 171.88,51.77 171.84,51.7
S$8528
  Bottom 0: 171.84,51.7 171.83,51.63
S$8529
  Bottom 0: 171.83,51.63 171.83,49.85
S$8530
  Bottom 0: 171.83,49.85 171.84,49.77
S$8531
  Bottom 0: 171.84,49.77 171.88,49.7
S$8532
  Bottom 0: 171.88,49.7 171.94,49.64
S$8533
  Bottom 0: 171.94,49.64 172.01,49.6
S$8534
  Bottom 0: 172.01,49.6 172.08,49.59
S$8535
  Bottom 0: 175.35,49.6 175.67,49.6
S$8536
  Bottom 0: 175.67,49.6 175.98,49.7
S$8537
  Bottom 0: 175.98,49.7 176.26,49.87
S$8538
  Bottom 0: 176.26,49.87 176.47,50.11
S$8539
  Bottom 0: 176.47,50.11 176.61,50.42
S$8540
  Bottom 0: 176.61,50.42 176.65,50.74
S$8541
  Bottom 0: 176.65,50.74 176.61,51.06
S$8542
  Bottom 0: 176.61,51.06 176.47,51.36
S$8543
  Bottom 0: 176.47,51.36 176.26,51.6
S$8544
  Bottom 0: 176.26,51.6 175.98,51.78
S$8545
  Bottom 0: 175.98,51.78 175.67,51.87
S$8546
  Bottom 0: 175.67,51.87 175.35,51.87
S$8547
  Bottom 0: 175.35,51.87 175.04,51.78
S$8548
  Bottom 0: 175.04,51.78 174.76,51.6
S$8549
  Bottom 0: 174.76,51.6 174.55,51.36
S$8550
  Bottom 0: 174.55,51.36 174.41,51.06
S$8551
  Bottom 0: 174.41,51.06 174.37,50.74
S$8552
  Bottom 0: 174.37,50.74 174.41,50.42
S$8553
  Bottom 0: 174.41,50.42 174.55,50.11
S$8554
  Bottom 0: 174.55,50.11 174.76,49.87
S$8555
  Bottom 0: 174.76,49.87 175.04,49.7
S$8556
  Bottom 0: 175.04,49.7 175.35,49.6
S$8557
  Bottom 0: 275.83,12.08 271.97,15.94
S$8558
  Bottom 0: 271.97,15.94 271.97,24.88
S$8559
  Bottom 0: 271.97,24.88 272.39,24.47
S$8560
  Bottom 0: 272.39,24.47 272.38,24.47
S$8561
  Bottom 0: 272.38,24.47 272.31,24.43
S$8562
  Bottom 0: 272.31,24.43 272.25,24.38
S$8563
  Bottom 0: 272.25,24.38 272.21,24.3
S$8564
  Bottom 0: 272.21,24.3 272.2,24.23
S$8565
  Bottom 0: 272.2,24.23 272.2,21.83
S$8566
  Bottom 0: 272.2,21.83 272.21,21.75
S$8567
  Bottom 0: 272.21,21.75 272.25,21.68
S$8568
  Bottom 0: 272.25,21.68 272.31,21.63
S$8569
  Bottom 0: 272.31,21.63 272.38,21.59
S$8570
  Bottom 0: 272.38,21.59 272.46,21.58
S$8571
  Bottom 0: 272.46,21.58 273.26,21.58
S$8572
  Bottom 0: 273.26,21.58 273.33,21.59
S$8573
  Bottom 0: 273.33,21.59 273.4,21.63
S$8574
  Bottom 0: 273.4,21.63 273.46,21.68
S$8575
  Bottom 0: 273.46,21.68 273.5,21.74
S$8576
  Bottom 0: 273.5,21.74 273.52,21.68
S$8577
  Bottom 0: 273.52,21.68 273.58,21.63
S$8578
  Bottom 0: 273.58,21.63 273.65,21.59
S$8579
  Bottom 0: 273.65,21.59 273.73,21.58
S$8580
  Bottom 0: 273.73,21.58 273.93,21.58
S$8581
  Bottom 0: 273.93,21.58 273.93,22.43
S$8582
  Bottom 0: 273.93,22.43 273.51,22.43
S$8583
  Bottom 0: 273.51,22.43 273.51,23.63
S$8584
  Bottom 0: 273.51,23.63 273.93,23.63
S$8585
  Bottom 0: 273.93,23.63 273.93,24.48
S$8586
  Bottom 0: 273.93,24.48 273.73,24.48
S$8587
  Bottom 0: 273.73,24.48 273.65,24.47
S$8588
  Bottom 0: 273.65,24.47 273.58,24.43
S$8589
  Bottom 0: 273.58,24.43 273.52,24.38
S$8590
  Bottom 0: 273.52,24.38 273.5,24.32
S$8591
  Bottom 0: 273.5,24.32 273.46,24.38
S$8592
  Bottom 0: 273.46,24.38 273.4,24.43
S$8593
  Bottom 0: 273.4,24.43 273.33,24.47
S$8594
  Bottom 0: 273.33,24.47 273.3,24.48
S$8595
  Bottom 0: 273.3,24.48 273.3,24.62
S$8596
  Bottom 0: 273.3,24.62 273.29,24.68
S$8597
  Bottom 0: 273.29,24.68 273.29,24.74
S$8598
  Bottom 0: 273.29,24.74 273.26,24.79
S$8599
  Bottom 0: 273.26,24.79 273.24,24.85
S$8600
  Bottom 0: 273.24,24.85 273.2,24.89
S$8601
  Bottom 0: 273.2,24.89 273.17,24.94
S$8602
  Bottom 0: 273.17,24.94 272.53,25.57
S$8603
  Bottom 0: 272.53,25.57 272.53,25.86
S$8604
  Bottom 0: 272.53,25.86 272.56,25.85
S$8605
  Bottom 0: 272.56,25.85 272.61,25.81
S$8606
  Bottom 0: 272.61,25.81 272.68,25.79
S$8607
  Bottom 0: 272.68,25.79 272.73,25.77
S$8608
  Bottom 0: 272.73,25.77 272.79,25.77
S$8609
  Bottom 0: 272.79,25.77 272.86,25.75
S$8610
  Bottom 0: 272.86,25.75 276.44,25.75
S$8611
  Bottom 0: 276.44,25.75 277.01,25.18
S$8612
  Bottom 0: 277.01,25.18 277.01,24.48
S$8613
  Bottom 0: 277.01,24.48 276.87,24.48
S$8614
  Bottom 0: 276.87,24.48 276.87,23.63
S$8615
  Bottom 0: 276.87,23.63 277.01,23.63
S$8616
  Bottom 0: 277.01,23.63 277.01,22.43
S$8617
  Bottom 0: 277.01,22.43 276.87,22.43
S$8618
  Bottom 0: 276.87,22.43 276.87,21.58
S$8619
  Bottom 0: 276.87,21.58 277.01,21.58
S$8620
  Bottom 0: 277.01,21.58 277.01,21.17
S$8621
  Bottom 0: 277.01,21.17 277.01,21.07
S$8622
  Bottom 0: 277.01,21.07 277.04,20.99
S$8623
  Bottom 0: 277.04,20.99 277.07,20.91
S$8624
  Bottom 0: 277.07,20.91 277.12,20.83
S$8625
  Bottom 0: 277.12,20.83 277.18,20.77
S$8626
  Bottom 0: 277.18,20.77 281.72,16.22
S$8627
  Bottom 0: 281.72,16.22 281.67,16.05
S$8628
  Bottom 0: 281.67,16.05 281.67,15.72
S$8629
  Bottom 0: 281.67,15.72 281.76,15.4
S$8630
  Bottom 0: 281.76,15.4 281.93,15.13
S$8631
  Bottom 0: 281.93,15.13 282.17,14.91
S$8632
  Bottom 0: 282.17,14.91 282.46,14.76
S$8633
  Bottom 0: 282.46,14.76 282.78,14.69
S$8634
  Bottom 0: 282.78,14.69 283.1,14.71
S$8635
  Bottom 0: 283.1,14.71 283.41,14.82
S$8636
  Bottom 0: 283.41,14.82 283.67,15.01
S$8637
  Bottom 0: 283.67,15.01 283.88,15.26
S$8638
  Bottom 0: 283.88,15.26 284,15.56
S$8639
  Bottom 0: 284,15.56 284.05,15.88
S$8640
  Bottom 0: 284.05,15.88 284,16.2
S$8641
  Bottom 0: 284,16.2 283.88,16.5
S$8642
  Bottom 0: 283.88,16.5 283.67,16.76
S$8643
  Bottom 0: 283.67,16.76 283.41,16.94
S$8644
  Bottom 0: 283.41,16.94 283.1,17.05
S$8645
  Bottom 0: 283.1,17.05 282.78,17.07
S$8646
  Bottom 0: 282.78,17.07 282.52,17.02
S$8647
  Bottom 0: 282.52,17.02 278.15,21.4
S$8648
  Bottom 0: 278.15,21.4 278.15,25.41
S$8649
  Bottom 0: 278.15,25.41 278.14,25.5
S$8650
  Bottom 0: 278.14,25.5 278.12,25.59
S$8651
  Bottom 0: 278.12,25.59 278.09,25.67
S$8652
  Bottom 0: 278.09,25.67 278.04,25.75
S$8653
  Bottom 0: 278.04,25.75 277.98,25.81
S$8654
  Bottom 0: 277.98,25.81 277.24,26.56
S$8655
  Bottom 0: 277.24,26.56 277.24,26.65
S$8656
  Bottom 0: 277.24,26.65 277.27,26.68
S$8657
  Bottom 0: 277.27,26.68 277.31,26.75
S$8658
  Bottom 0: 277.31,26.75 277.32,26.83
S$8659
  Bottom 0: 277.32,26.83 277.32,29.02
S$8660
  Bottom 0: 277.32,29.02 280.44,25.9
S$8661
  Bottom 0: 280.44,25.9 280.44,25.89
S$8662
  Bottom 0: 280.44,25.89 280.45,25.89
S$8663
  Bottom 0: 280.45,25.89 280.98,25.37
S$8664
  Bottom 0: 280.98,25.37 280.98,23.91
S$8665
  Bottom 0: 280.98,23.91 280.73,23.78
S$8666
  Bottom 0: 280.73,23.78 280.5,23.56
S$8667
  Bottom 0: 280.5,23.56 280.32,23.28
S$8668
  Bottom 0: 280.32,23.28 280.24,22.97
S$8669
  Bottom 0: 280.24,22.97 280.24,22.64
S$8670
  Bottom 0: 280.24,22.64 280.32,22.33
S$8671
  Bottom 0: 280.32,22.33 280.5,22.05
S$8672
  Bottom 0: 280.5,22.05 280.73,21.83
S$8673
  Bottom 0: 280.73,21.83 281.01,21.68
S$8674
  Bottom 0: 281.01,21.68 281.34,21.62
S$8675
  Bottom 0: 281.34,21.62 281.66,21.64
S$8676
  Bottom 0: 281.66,21.64 281.96,21.75
S$8677
  Bottom 0: 281.96,21.75 282.23,21.93
S$8678
  Bottom 0: 282.23,21.93 282.44,22.19
S$8679
  Bottom 0: 282.44,22.19 282.57,22.49
S$8680
  Bottom 0: 282.57,22.49 282.61,22.81
S$8681
  Bottom 0: 282.61,22.81 282.57,23.13
S$8682
  Bottom 0: 282.57,23.13 282.44,23.43
S$8683
  Bottom 0: 282.44,23.43 282.23,23.68
S$8684
  Bottom 0: 282.23,23.68 281.96,23.87
S$8685
  Bottom 0: 281.96,23.87 281.86,23.9
S$8686
  Bottom 0: 281.86,23.9 281.86,25.55
S$8687
  Bottom 0: 281.86,25.55 281.86,25.62
S$8688
  Bottom 0: 281.86,25.62 281.84,25.69
S$8689
  Bottom 0: 281.84,25.69 281.81,25.75
S$8690
  Bottom 0: 281.81,25.75 281.77,25.81
S$8691
  Bottom 0: 281.77,25.81 281.73,25.86
S$8692
  Bottom 0: 281.73,25.86 281.39,26.2
S$8693
  Bottom 0: 281.39,26.2 284.52,29.34
S$8694
  Bottom 0: 284.52,29.34 284.58,29.31
S$8695
  Bottom 0: 284.58,29.31 284.9,29.24
S$8696
  Bottom 0: 284.9,29.24 285.23,29.26
S$8697
  Bottom 0: 285.23,29.26 285.53,29.37
S$8698
  Bottom 0: 285.53,29.37 285.8,29.56
S$8699
  Bottom 0: 285.8,29.56 286.01,29.81
S$8700
  Bottom 0: 286.01,29.81 286.13,30.11
S$8701
  Bottom 0: 286.13,30.11 286.18,30.43
S$8702
  Bottom 0: 286.18,30.43 286.13,30.75
S$8703
  Bottom 0: 286.13,30.75 286.01,31.05
S$8704
  Bottom 0: 286.01,31.05 285.8,31.3
S$8705
  Bottom 0: 285.8,31.3 285.53,31.49
S$8706
  Bottom 0: 285.53,31.49 285.23,31.6
S$8707
  Bottom 0: 285.23,31.6 284.9,31.62
S$8708
  Bottom 0: 284.9,31.62 284.58,31.55
S$8709
  Bottom 0: 284.58,31.55 284.3,31.41
S$8710
  Bottom 0: 284.3,31.41 284.06,31.18
S$8711
  Bottom 0: 284.06,31.18 283.89,30.91
S$8712
  Bottom 0: 283.89,30.91 283.8,30.59
S$8713
  Bottom 0: 283.8,30.59 283.8,30.27
S$8714
  Bottom 0: 283.8,30.27 283.89,29.96
S$8715
  Bottom 0: 283.89,29.96 280.76,26.84
S$8716
  Bottom 0: 280.76,26.84 277.69,29.91
S$8717
  Bottom 0: 277.69,29.91 277.63,29.95
S$8718
  Bottom 0: 277.63,29.95 277.57,29.99
S$8719
  Bottom 0: 277.57,29.99 277.51,30.02
S$8720
  Bottom 0: 277.51,30.02 277.44,30.04
S$8721
  Bottom 0: 277.44,30.04 277.37,30.04
S$8722
  Bottom 0: 277.37,30.04 272.2,30.04
S$8723
  Bottom 0: 272.2,30.04 272.12,30.04
S$8724
  Bottom 0: 272.12,30.04 272.06,30.02
S$8725
  Bottom 0: 272.06,30.02 272,30
S$8726
  Bottom 0: 272,30 271.97,29.98
S$8727
  Bottom 0: 271.97,29.98 271.97,39.45
S$8728
  Bottom 0: 271.97,39.45 283.81,51.29
S$8729
  Bottom 0: 283.81,51.29 284.01,51.27
S$8730
  Bottom 0: 284.01,51.27 284.25,51.34
S$8731
  Bottom 0: 284.25,51.34 284.46,51.49
S$8732
  Bottom 0: 284.46,51.49 284.59,51.7
S$8733
  Bottom 0: 284.59,51.7 284.63,51.95
S$8734
  Bottom 0: 284.63,51.95 284.59,52.2
S$8735
  Bottom 0: 284.59,52.2 284.46,52.42
S$8736
  Bottom 0: 284.46,52.42 284.3,52.54
S$8737
  Bottom 0: 284.3,52.54 284.3,56.9
S$8738
  Bottom 0: 284.3,56.9 284.29,56.97
S$8739
  Bottom 0: 284.29,56.97 284.27,57.03
S$8740
  Bottom 0: 284.27,57.03 284.25,57.1
S$8741
  Bottom 0: 284.25,57.1 284.21,57.16
S$8742
  Bottom 0: 284.21,57.16 284.17,57.21
S$8743
  Bottom 0: 284.17,57.21 274.05,67.33
S$8744
  Bottom 0: 274.05,67.33 275.62,67.33
S$8745
  Bottom 0: 275.62,67.33 286.54,56.41
S$8746
  Bottom 0: 286.54,56.41 286.54,56.24
S$8747
  Bottom 0: 286.54,56.24 286.63,56.01
S$8748
  Bottom 0: 286.63,56.01 286.8,55.82
S$8749
  Bottom 0: 286.8,55.82 287.03,55.71
S$8750
  Bottom 0: 287.03,55.71 287.28,55.69
S$8751
  Bottom 0: 287.28,55.69 287.52,55.76
S$8752
  Bottom 0: 287.52,55.76 287.72,55.91
S$8753
  Bottom 0: 287.72,55.91 287.86,56.12
S$8754
  Bottom 0: 287.86,56.12 287.9,56.37
S$8755
  Bottom 0: 287.9,56.37 287.86,56.62
S$8756
  Bottom 0: 287.86,56.62 287.72,56.83
S$8757
  Bottom 0: 287.72,56.83 287.52,56.98
S$8758
  Bottom 0: 287.52,56.98 287.28,57.05
S$8759
  Bottom 0: 287.28,57.05 287.17,57.04
S$8760
  Bottom 0: 287.17,57.04 276.14,68.08
S$8761
  Bottom 0: 276.14,68.08 276.75,68.08
S$8762
  Bottom 0: 276.75,68.08 276.76,68.04
S$8763
  Bottom 0: 276.76,68.04 276.93,67.77
S$8764
  Bottom 0: 276.93,67.77 277.17,67.54
S$8765
  Bottom 0: 277.17,67.54 277.45,67.39
S$8766
  Bottom 0: 277.45,67.39 277.77,67.33
S$8767
  Bottom 0: 277.77,67.33 278.1,67.35
S$8768
  Bottom 0: 278.1,67.35 278.4,67.45
S$8769
  Bottom 0: 278.4,67.45 278.67,67.64
S$8770
  Bottom 0: 278.67,67.64 278.88,67.89
S$8771
  Bottom 0: 278.88,67.89 279.01,68.2
S$8772
  Bottom 0: 279.01,68.2 279.05,68.52
S$8773
  Bottom 0: 279.05,68.52 279.01,68.84
S$8774
  Bottom 0: 279.01,68.84 278.88,69.14
S$8775
  Bottom 0: 278.88,69.14 278.67,69.39
S$8776
  Bottom 0: 278.67,69.39 278.4,69.58
S$8777
  Bottom 0: 278.4,69.58 278.1,69.69
S$8778
  Bottom 0: 278.1,69.69 277.77,69.7
S$8779
  Bottom 0: 277.77,69.7 277.45,69.64
S$8780
  Bottom 0: 277.45,69.64 277.17,69.49
S$8781
  Bottom 0: 277.17,69.49 276.93,69.27
S$8782
  Bottom 0: 276.93,69.27 276.76,68.99
S$8783
  Bottom 0: 276.76,68.99 276.75,68.96
S$8784
  Bottom 0: 276.75,68.96 271.54,68.96
S$8785
  Bottom 0: 271.54,68.96 271.72,69.16
S$8786
  Bottom 0: 271.72,69.16 271.86,69.47
S$8787
  Bottom 0: 271.86,69.47 271.9,69.79
S$8788
  Bottom 0: 271.9,69.79 271.86,70.09
S$8789
  Bottom 0: 271.86,70.09 276.59,74.81
S$8790
  Bottom 0: 276.59,74.81 276.65,74.88
S$8791
  Bottom 0: 276.65,74.88 276.7,74.96
S$8792
  Bottom 0: 276.7,74.96 276.74,75.04
S$8793
  Bottom 0: 276.74,75.04 276.75,75.13
S$8794
  Bottom 0: 276.75,75.13 276.76,75.22
S$8795
  Bottom 0: 276.76,75.22 276.76,76.24
S$8796
  Bottom 0: 276.76,76.24 282.44,76.24
S$8797
  Bottom 0: 282.44,76.24 282.44,76.21
S$8798
  Bottom 0: 282.44,76.21 282.46,76.14
S$8799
